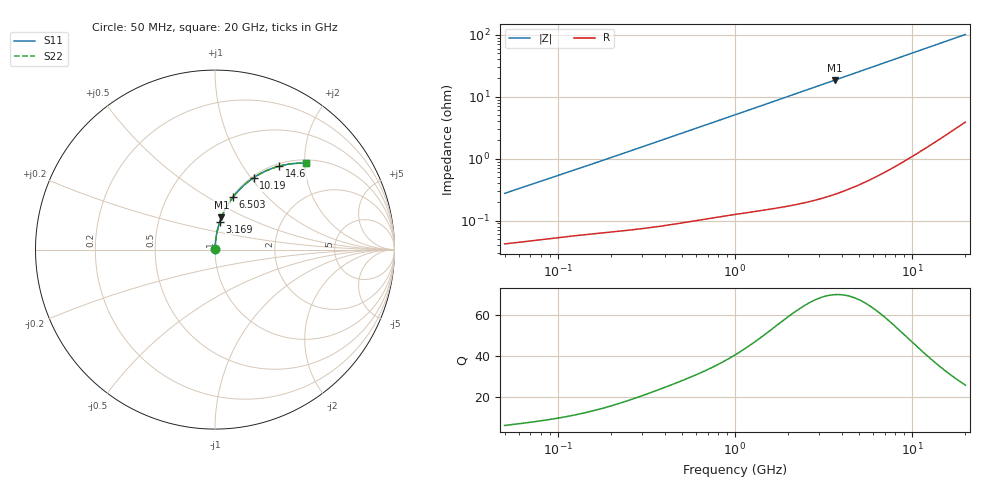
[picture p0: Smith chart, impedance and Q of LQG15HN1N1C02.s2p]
!Murata Part Number: LQG15HN1N1C02
!These Parameters are Measured in Series Mode Connection
!  o--[Z]--o
!Port1  Port2
!  o-------o
!Freq. Start=50[MHz] Stop=20[GHz], 401[Steps]
# Hz S RI R 50
!Freq.(Hz) S11(Real) S11(Imag) S21(Real) S21(Imag) S12(Real) S12(Imag) S22(Real) S22(Imag)
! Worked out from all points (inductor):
!   401 points, 50 MHz to 20 GHz, reference 50 ohm
!   read as one part in series: L = 859 pH near 51.52 MHz
!   highest Q = 69.8 at 3.681 GHz (marker M1), where L = 806 pH
!   S11 on the Smith chart (normalised r, x): 50 MHz: 1.00, +0.01; 3.169 GHz: 1.00, +0.32; 6.503 GHz: 1.01, +0.66; 10.19 GHz: 1.02, +1.03; 14.6 GHz: 1.04, +1.48; 20 GHz: 1.08, +2.02
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5e7  0.000428 0.00272  0.9996 -0.00272  0.9996 -0.00272  0.000428 0.00272
5.152053e7  0.000432 0.0028  0.9996 -0.0028  0.9996 -0.0028  0.000432 0.0028
1.364002e8  0.000637 0.00717  0.9994 -0.00717  0.9994 -0.00717  0.000637 0.00717
3.721004e8  0.00117 0.0192  0.9988 -0.0192  0.9988 -0.0192  0.00117 0.0192
6.380365e8  0.00209 0.0326  0.9979 -0.0326  0.9979 -0.0326  0.00209 0.0326
1e9  0.00384 0.0507  0.9962 -0.0507  0.9962 -0.0507  0.00384 0.0507
1.329223e9  0.00595 0.0671  0.9941 -0.0671  0.9941 -0.0671  0.00595 0.0671
1.714689e9  0.00907 0.0861  0.9909 -0.0861  0.9909 -0.0861  0.00907 0.0861
2.179053e9  0.0138 0.1088  0.9862 -0.1088  0.9862 -0.1088  0.0138 0.1088
2.728004e9  0.0207 0.1351  0.9793 -0.1351  0.9793 -0.1351  0.0207 0.1351
3.168813e9  0.0273 0.1557  0.9727 -0.1557  0.9727 -0.1557  0.0273 0.1557
3.680849e9  0.036 0.1792  0.964 -0.1792  0.964 -0.1792  0.036 0.1792
4.966507e9  0.0625 0.2348  0.9375 -0.2348  0.9375 -0.2348  0.0625 0.2348
6.503449e9  0.1016 0.2941  0.8984 -0.2941  0.8984 -0.2941  0.1016 0.2941
7.442007e9  0.1285 0.326  0.8715 -0.326  0.8715 -0.326  0.1285 0.326
8.774992e9  0.1695 0.3656  0.8305 -0.3656  0.8305 -0.3656  0.1695 0.3656
1.019291e10  0.2152 0.4003  0.7848 -0.4003  0.7848 -0.4003  0.2152 0.4003
1.220001e10  0.2809 0.4371  0.7191 -0.4371  0.7191 -0.4371  0.2809 0.4371
1.460232e10  0.3572 0.4649  0.6428 -0.4649  0.6428 -0.4649  0.3572 0.4649
1.721783e10  0.4338 0.4791  0.5662 -0.4791  0.5662 -0.4791  0.4338 0.4791
1.940974e10  0.4915 0.4815  0.5085 -0.4815  0.5085 -0.4815  0.4915 0.4815
2e10  0.5059 0.4811  0.4941 -0.4811  0.4941 -0.4811  0.5059 0.4811
